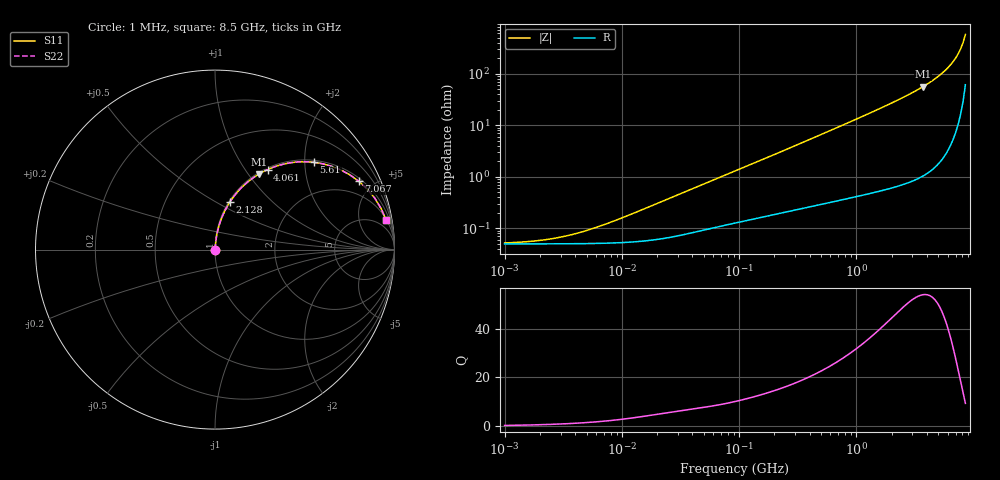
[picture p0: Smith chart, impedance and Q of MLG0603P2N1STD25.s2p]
! S-Parameter Data Generated by TDK Corporation
! Copyright(C) 2025 TDK Corporation.
! All Rights Reserved.
! TDK P/N: MLG0603P2N1STD25 (SMD / SMT Inductor (Coil))
! Property: L=2.1nH at 500MHz
! Size(LxWxT): 0.6x0.3x0.3mm
! Model Type: s2p (Touchstone File Format Version 1.0)
! Frequency: DC=Yes Start=1MHz Stop=8500MHz 198points Log-sweep
! Model Generated on Feb. 6, 2025
! Terms and conditions regarding TDK Simulation Models:
! 1)This simulation model is being provided solely for informational
!  purposes. Please refer to the specifications of the products in
!  terms of detailed characteristics of such products.
! 2)In no event shall TDK Corporation of any of its subsidiaries be
!  liable for any loss or damage arising, directly or indirectly,
!  from any information contained in this simulation model, including,
!  but not limited to loss or damages arising from any inaccuracies,
!  omissions or errors in connection with such information.
! 3)Any and all copyrights on this simulation model are owned by
!  TDK Corporation.  Duplication or redistribution of this simulation
!  model without prior written permission from TDK Corporation
!  is prohibited.
! 4)This simulation model is subject to any modification or change
!  without any prior notice.
! 5)Neither TDK Corporation nor any of its subsidiaries shall make any
!  warranty, express or implied, including but not limited to the
!  correctness, implied warranties of merchantability and fitness for
!  a particular purpose with respect to this simulation models.
! 6)The use of this simulation model shall be deemed to have consented
!  to the terms and conditions hereof.
! Port Assignments:
!  1 ---@@@--- 2
! Applicable Conditions:
!  Temperature = 25 degC
!  DC Bias Current = 0 A
!  Small Signal Operation
# Hz S MA R 50
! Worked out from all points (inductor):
!   197 points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, 1 MHz to 8.5 GHz, reference 50 ohm
!   read as one part in series: L = 2.39 nH near 11.03 MHz
!   highest Q = 54 at 3.703 GHz (marker M1), where L = 2.41 nH
!   S11 on the Smith chart (normalised r, x): 1 MHz: 1.00, +0.00; 2.128 GHz: 1.01, +0.58; 4.061 GHz: 1.02, +1.28; 5.61 GHz: 1.05, +2.22; 7.067 GHz: 1.15, +4.11; 8.5 GHz: 2, +11
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1000000  0.0005224 16.8  0.9995 -0.0  0.9995 -0.0  0.0005224 16.8
1586648  0.000555 25.6  0.9995 -0.0  0.9995 -0.0  0.000555 25.6
2295435  0.0006096 34.6  0.9995 -0.0  0.9995 -0.0  0.0006096 34.6
3320851  0.0007104 44.9  0.9995 -0.0  0.9995 -0.0  0.0007104 44.9
4587603  0.0008579 53.8  0.9995 -0.0  0.9995 -0.0  0.0008579 53.8
8360083  0.001363 67.4  0.9995 -0.1  0.9995 -0.1  0.001363 67.4
2.10461e7  0.003193 78.6  0.9994 -0.2  0.9994 -0.2  0.003193 78.6
9.219544e7  0.01287 83.6  0.9987 -0.7  0.9987 -0.7  0.01287 83.6
4.229561e8  0.05581 84.1  0.9958 -3.2  0.9958 -3.2  0.05581 84.1
9.708683e8  0.1261 80.9  0.988 -7.2  0.988 -7.2  0.1261 80.9
1.940355e9  0.2512 74.1  0.9622 -14.5  0.9622 -14.5  0.2512 74.1
2.128028e9  0.2757 72.7  0.9552 -16.0  0.9552 -16.0  0.2757 72.7
2.939772e9  0.383 66.4  0.9164 -22.5  0.9164 -22.5  0.383 66.4
3.703002e9  0.4854 59.9  0.8653 -29.0  0.8653 -29.0  0.4854 59.9
4.061159e9  0.5336 56.7  0.8359 -32.2  0.8359 -32.2  0.5336 56.7
4.884749e9  0.6431 48.9  0.7532 -40.0  0.7532 -40.0  0.6431 48.9
5.610304e9  0.7348 41.4  0.6621 -47.3  0.6621 -47.3  0.7348 41.4
6.44363e9  0.8286 32.5  0.5368 -55.9  0.5368 -55.9  0.8286 32.5
7.066863e9  0.8866 25.5  0.4311 -62.4  0.4311 -62.4  0.8866 25.5
7.750377e9  0.935 17.9  0.3073 -69.0  0.3073 -69.0  0.935 17.9
8.116539e9  0.9538 13.8  0.2394 -72.0  0.2394 -72.0  0.9538 13.8
8.5e9  0.968 9.6  0.1685 -74.3  0.1685 -74.3  0.968 9.6
